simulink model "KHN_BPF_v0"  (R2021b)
settings: Solver=VariableStepAuto  StartTime=0.0  StopTime=0.5  MaxStep=1e-4  RelTol=1e-3
libraries: fl_lib x19, nesl_utility x4

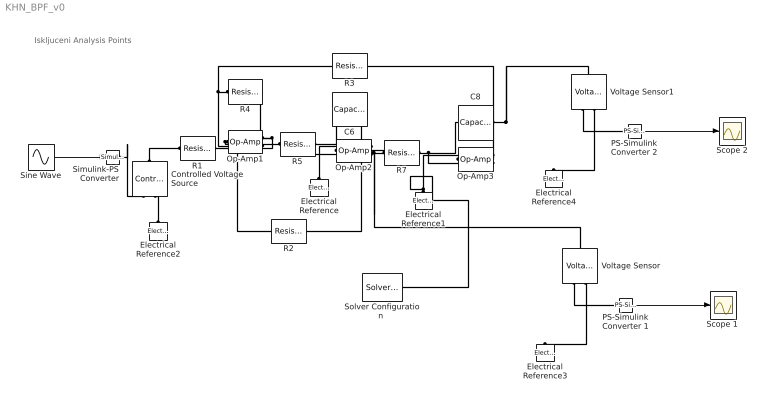
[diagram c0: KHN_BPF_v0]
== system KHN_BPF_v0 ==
  note: Iskljuceni Analysis Points
  C6 : fl_lib/Electrical/Electrical Elements/Capacitor  c=1e-6 F  r=1e-6 Ohm  g=0 1/Ohm  i_specify=off  i_priority=None  i=0 A  i_nominal_specify=off  i_nominal_unit=A  i_nominal_value=1  v_specify=off  v_priority=None  v=0 V  v_nominal_specify=off  v_nominal_unit=V  v_nominal_value=1  vc_specify=off  vc_priority=High  vc=0 V  vc_nominal_specify=off  vc_nominal_unit=V  vc_nominal_value=1
  C8 : fl_lib/Electrical/Electrical Elements/Capacitor  c=1e-6 F  r=1e-6 Ohm  g=0 1/Ohm  i_specify=off  i_priority=None  i=0 A  i_nominal_specify=off  i_nominal_unit=A  i_nominal_value=1  v_specify=off  v_priority=None  v=0 V  v_nominal_specify=off  v_nominal_unit=V  v_nominal_value=1  vc_specify=off  vc_priority=High  vc=0 V  vc_nominal_specify=off  vc_nominal_unit=V  vc_nominal_value=1
  "Controlled Voltage Source " : fl_lib/Electrical/Electrical Sources/Controlled Voltage Source
  Electrical Reference{,1..4} (5 alike) : fl_lib/Electrical/Electrical Elements/Electrical Reference
  Op-Amp1 : fl_lib/Electrical/Electrical Elements/Op-Amp  outI_specify=off  outI_priority=None  outI=0 A  outI_nominal_specify=off  outI_nominal_unit=A  outI_nominal_value=1
  Op-Amp2 : fl_lib/Electrical/Electrical Elements/Op-Amp  outI_specify=off  outI_priority=None  outI=0 A  outI_nominal_specify=off  outI_nominal_unit=A  outI_nominal_value=1
  Op-Amp3 : fl_lib/Electrical/Electrical Elements/Op-Amp  outI_specify=off  outI_priority=None  outI=0 A  outI_nominal_specify=off  outI_nominal_unit=A  outI_nominal_value=1
  PS-Simulink Converter 1 : nesl_utility/PS-Simulink Converter  PhysicalDomain=network_engine_domain  SubClassName=ps_output  LeftPortType=input  RightPortType=output  PseudoPeriodic=off  Frequencies=[]  Unit=inherit  AffineConversion=off
  PS-Simulink Converter 2 : nesl_utility/PS-Simulink Converter  PhysicalDomain=network_engine_domain  SubClassName=ps_output  LeftPortType=input  RightPortType=output  PseudoPeriodic=off  Frequencies=[]  Unit=inherit  AffineConversion=off
  R{1,3..5,7} (5 alike) : fl_lib/Electrical/Electrical Elements/Resistor  R=1 kOhm  i_specify=off  i_priority=None  i=0 A  i_nominal_specify=off  i_nominal_unit=A  i_nominal_value=1  v_specify=off  v_priority=None  v=0 V  v_nominal_specify=off  v_nominal_unit=V  v_nominal_value=1
  R2 : fl_lib/Electrical/Electrical Elements/Resistor  R=2 kOhm  i_specify=off  i_priority=None  i=0 A  i_nominal_specify=off  i_nominal_unit=A  i_nominal_value=1  v_specify=off  v_priority=None  v=0 V  v_nominal_specify=off  v_nominal_unit=V  v_nominal_value=1
  "Scope 1 " : Scope
  Scope 2 : Scope
  Simulink-PS Converter : nesl_utility/Simulink-PS Converter  PhysicalDomain=network_engine_domain  SubClassName=ps_input  LeftPortType=input  RightPortType=output  PseudoPeriodic=off  Frequencies=[]  NoiseDistribution=none  NoiseParameters=[]  Unit=1  AffineConversion=off  FilteringAndDerivatives=provide  SimscapeFilterOrder=1  InputFilterTimeConstant=0.001  UdotUserProvided=0
  Sine Wave : Sin  Frequency=1000  SampleTime=0
  "Solver Configuration " : nesl_utility/Solver Configuration  PhysicalDomain=network_engine_domain  SubClassName=solver  LeftPortType=input  RightPortType=generic  Tones=[]  Harmonics=[]  SimulateNoise=off  Profile=off  UseLocalSampling=off  EnableSwitchedLinearOptims=on  FrequencyDomain=off  UseCCode=off  RelTol=0.001  AbsTol=1e-06  MinStep=1e-09  ToWorkspace=off  RevertToSquareIcSolve=off  NumHomotopyIterations=100  PhasorMode=off  PhasorModeNumHarmonics=1  DoDC=on  ResidualTolerance=1e-09  UseLocalSolver=off  LocalSolverChoice=NE_BACKWARD_EULER_ADVANCER  LocalSolverSampleTime=0.001  DoFixedCost=off  MaxNonlinIter=3  MaxModeIter=2  ComputeImpulses=off  ImpulseIterations=2  LinearAlgebra=auto  EquationFormulation=NE_TIME_EF  DelaysMemoryBudget=1024  AutomaticFiltering=on  FilteringTimeConstant=0.001  PartitionStorageMethod=AS_NEEDED  PartitionMemoryBudget=1024  PartitionMethod=ROBUST
  Voltage Sensor : fl_lib/Electrical/Electrical Sensors/Voltage Sensor
  Voltage Sensor1 : fl_lib/Electrical/Electrical Sensors/Voltage Sensor
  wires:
  Sine Wave/1 -> Simulink-PS Converter/1
  PS-Simulink Converter 1/1 -> "Scope 1 "/1
  PS-Simulink Converter 2/1 -> Scope 2/1
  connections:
  R5/RConn1 -- C6/LConn1 -- Op-Amp2/LConn2
  R7/RConn1 -- C8/LConn1 -- Op-Amp3/LConn2
  R7/LConn1 -- R2/RConn1 -- Voltage Sensor/LConn1 -- C6/RConn1 -- Op-Amp2/RConn1
  C8/RConn1 -- Voltage Sensor1/LConn1 -- R3/RConn1 -- Op-Amp3/RConn1
  Op-Amp1/RConn1 -- R4/RConn1 -- R5/LConn1
  R4/LConn1 -- Op-Amp1/LConn2 -- R3/LConn1
  Op-Amp1/LConn1 -- R2/LConn1 -- R1/RConn1
  Electrical Reference/LConn1 -- Op-Amp2/LConn1
  Electrical Reference1/LConn1 -- "Solver Configuration "/RConn1 -- Op-Amp3/LConn1
  "Controlled Voltage Source "/RConn1 -- Simulink-PS Converter/RConn1
  Electrical Reference2/LConn1 -- "Controlled Voltage Source "/RConn2
  "Controlled Voltage Source "/LConn1 -- R1/LConn1
  Voltage Sensor/RConn1 -- PS-Simulink Converter 1/LConn1
  Voltage Sensor/RConn2 -- Electrical Reference3/LConn1
  Voltage Sensor1/RConn2 -- Electrical Reference4/LConn1
  Voltage Sensor1/RConn1 -- PS-Simulink Converter 2/LConn1
